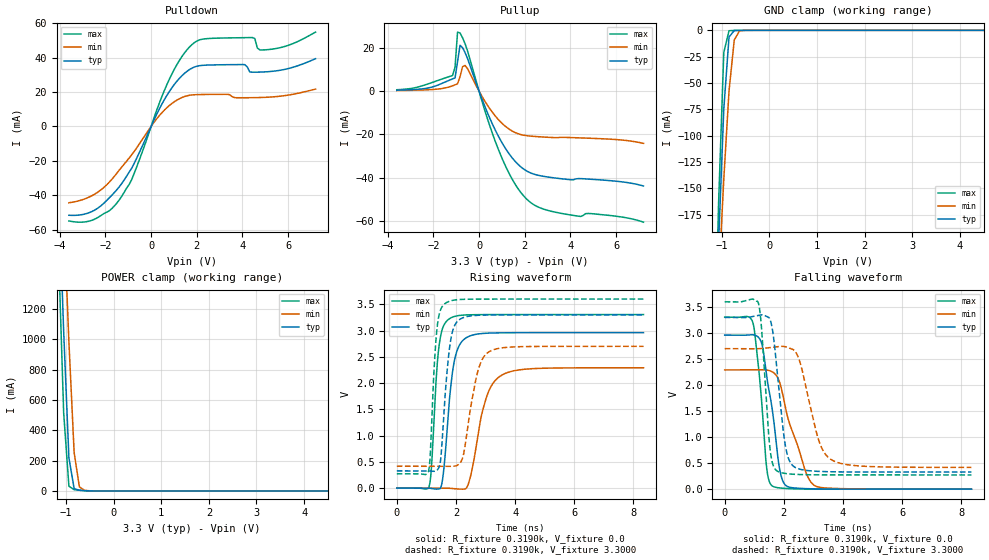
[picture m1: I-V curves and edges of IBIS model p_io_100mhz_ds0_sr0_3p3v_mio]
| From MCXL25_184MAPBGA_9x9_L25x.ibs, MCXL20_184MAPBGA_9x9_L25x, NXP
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[Model] p_io_100mhz_ds0_sr0_3p3v_mio
|   Model p_io_100mhz_ds0_sr0_3p3v_mio
| This model was characterised for following simulation conditions:
| External (pad) voltage:
|   - Typ: 3.3V,   - Min: 2.7V,   - Max: 3.6V
| Library cells for typ/min/max conditions are connected as defined below:
|  pad - External Pad
|  ipp_do_lv - Core Input
|  ipp_obe_lv - Output Buffer Enable
|  IOGC - NC
|  REFH3V3 - REFH3V3
|  REFL3V3 - REFL3V3
|  ZI - NC
|  abut_ncal_vddio[1] - vddio
|  abut_ncal_vddio[2] - vddio
|  abut_ncal_vddio[3] - vssio
|  abut_ncal_vddio[4] - vddio
|  abut_ncal_vddio[5] - vddio
|  abut_ncal_vddio[6] - vssio
|  abut_pcal_vddio[1] - vssio
|  abut_pcal_vddio[2] - vssio
|  abut_pcal_vddio[3] - vddio
|  abut_pcal_vddio[4] - vssio
|  abut_pcal_vddio[5] - vssio
|  abut_pcal_vddio[6] - vddio
|  ipp_do_1p8v - ipp_do_1p8v
|  ipp_dse_lv - 0
|  ipp_eftd_lv - NC
|  ipp_ina_mux_vddio - NC
|  ipp_ina_mux_vddio[0] - NC
|  ipp_ina_mux_vddio[1] - NC
|  ipp_ina_r0_vddio - NC
|  ipp_ina_r0a_vddio - NC
|  ipp_ina_r0b_vddio - NC
|  ipp_ina_r0c_vddio - NC
|  ipp_ina_r0d_vddio - NC
|  ipp_ina_r0e_vddio - NC
|  ipp_ina_r0f_vddio - NC
|  ipp_ina_r300_vddio - NC
|  ipp_ina_r300a_vddio - NC
|  ipp_ina_r300b_vddio - NC
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Model_type I/O
Polarity   Non-Inverting
Enable   Active-High
Vinl =   0.9900V
Vinh =   2.3100V
Vmeas =  1.6500V
Cref =   30.0000pF
Rref =   1.0000M
Vref =   3.3000V
C_comp   1.3235pF   1.2640pF   1.4076pF
|C_comp_pullup   0.6739pF   0.7056pF   0.6519pF
|C_comp_pulldown   0.5816pF   0.6344pF   0.5434pF
[Model Spec]
| variable   typ   min   max
Vinh   2.3100V   1.8900V   2.5200V
Vinl   0.9900V   0.8100V   1.0800V
[Temperature Range]   25.0000   0.1250k   -40.0000
[Voltage Range]   3.3000V   2.7000V   3.6000V
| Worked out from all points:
|   slope of the pulldown table from 0 to 0.495 V, typ, clamps not added: 36.6 ohm
|   slope of the pullup table from 0 to 0.495 V, typ, clamps not added: 37.7 ohm
|   GND clamp passes 1 mA (typ) near -0.75 V on its own axis
|   POWER clamp passes 1 mA (typ) near -0.55 V on its own axis
|   rising waveform, R_fixture 0.3190k, V_fixture 0.0: 20-80 % time 299ps typ, 517ps min, 214ps max; typ from 0 V to 2.96 V
|   rising waveform, R_fixture 0.3190k, V_fixture 3.3000: 20-80 % time 255ps typ, 423ps min, 184ps max; typ from 0.328 V to 3.3 V
|   falling waveform, R_fixture 0.3190k, V_fixture 0.0: 20-80 % time 427ps typ, 707ps min, 290ps max; typ from 2.96 V to 0 V
|   falling waveform, R_fixture 0.3190k, V_fixture 3.3000: 20-80 % time 330ps typ, 583ps min, 237ps max; typ from 3.3 V to 0.329 V
[Pulldown]
|Voltage   I(typ)   I(min)   I(max)
-3.6V     -51.52mA   -44.27mA   -54.81mA
-2.5V     -48.75mA   -39.51mA   -53.96mA
-1.4V     -35.12mA   -25.45mA   -42.73mA
-850mV    -24.27mA   -16.41mA   -30.84mA
800mV     20.29mA    12.16mA    27.43mA
1.35V     29.44mA    16.78mA    40.57mA
1.9V      34.5mA     18.39mA    48.67mA
4.1V      35.87mA    16.66mA    51.51mA
4.43V     31.5mA     16.69mA    51.59mA
4.65V     31.5mA     16.75mA    45.53mA
5.09V     31.75mA    16.96mA    44.55mA
7.2V      39.3mA     21.67mA    54.74mA
[Pullup]
|Voltage   I(typ)   I(min)   I(max)
-3.6V     391.8uA    234.9uA    605.7uA
-1.16V    5.604mA    2.419mA    7.14mA
-1.05V    6.055mA    2.871mA    11mA
-940mV    13.56mA    3.339mA    27.24mA
-830mV    21.15mA    6.685mA    26.82mA
-720mV    20.05mA    11.26mA    24.61mA
-610mV    17.74mA    11.81mA    21.86mA
820mV     -20.29mA   -12.86mA   -26.23mA
1.48V     -31.23mA   -18.63mA   -41.23mA
2.03V     -36.57mA   -20.53mA   -49.31mA
3.46V     -40.33mA   -21.49mA   -56.22mA
7.2V      -43.87mA   -24.17mA   -60.58mA
[GND_clamp]
|Voltage   I(typ)   I(min)   I(max)
-3.6V     -4.134A    -3.035A    -5.609A
-1.18V    -349.4mA   -343.6mA   -365.7mA
-1.07V    -202.9mA   -239.3mA   -165.2mA
-960mV    -74.83mA   -141.5mA   -21.03mA
-850mV    -6.389mA   -57.64mA   -383.3uA
-740mV    -222.1uA   -9.174mA   -124.1uA
-630mV    -55.93uA   -558.9uA   -58.07uA
7.2V      0A         0A         0A
[POWER_clamp]
|Voltage   I(typ)   I(min)   I(max)
-3.6V     24.54A     22.33A     26.93A
-1.16V    2.046A     2.721A     1.599A
-1.05V    1.052A     1.847A     514.4mA
-940mV    218.6mA    981.8mA    31.16mA
-830mV    15.1mA     252.4mA    8.462mA
-720mV    4.281mA    26.81mA    4.453mA
-610mV    1.717mA    3.626mA    1.66mA
7.2V      0A         0A         0A
[Ramp]
| variable   typ   min   max
dV/dt_r  1.7763/0.2988n   1.3750/0.5172n   1.9832/0.2140n
dV/dt_f  1.7829/0.3304n   1.3692/0.5829n   1.9962/0.2366n
R_load = 0.3190k
[Rising Waveform]
R_fixture= 0.3190k
V_fixture= 0.0
V_fixture_min= 0.0
V_fixture_max= 0.0
|time   V(typ)   V(min)   V(max)
0s        2.902nV    250nV      9.459nV
1.086ns   -976.7uV   -29.66uV   18.83mV
1.414ns   -15.5mV    651.1uV    2.638V
1.567ns   247.8mV    1.45mV     3.071V
1.766ns   1.596V     -2.144mV   3.22V
2.173ns   2.772V     -19.8mV    3.292V
2.455ns   2.894V     144.2mV    3.3V
3.05ns    2.95V      1.761V     3.304V
3.542ns   2.957V     2.149V     3.305V
8.34ns    2.961V     2.292V     3.305V
[Rising Waveform]
R_fixture= 0.3190k
V_fixture= 3.3000
V_fixture_min= 2.7000
V_fixture_max= 3.6000
|time   V(typ)   V(min)   V(max)
0s        328.4mV    417.4mV    273mV
1.073ns   327.9mV    417.3mV    324.4mV
1.356ns   339mV      417.7mV    3.019V
1.484ns   549.3mV    418.3mV    3.402V
1.64ns    1.817V     417.6mV    3.518V
1.974ns   3.118V     421.1mV    3.583V
2.25ns    3.247V     626.3mV    3.595V
2.767ns   3.292V     2.277V     3.599V
3.119ns   3.297V     2.597V     3.6V
8.34ns    3.3V       2.7V       3.6V
[Falling Waveform]
R_fixture= 0.3190k
V_fixture= 0.0
V_fixture_min= 0.0
V_fixture_max= 0.0
|time   V(typ)   V(min)   V(max)
0s        2.961V     2.292V     3.305V
954.1ps   2.967V     2.291V     3.197V
1.243ns   2.815V     2.294V     1.731V
1.42ns    2.166V     2.29V      403.1mV
1.604ns   1.548V     2.256V     63.43mV
1.828ns   486.1mV    2.1V       25.24mV
1.982ns   134.6mV    1.766V     16.49mV
2.726ns   10.64mV    351.6mV    2.556mV
3.05ns    5.57mV     66.35mV    1.221mV
8.34ns    83.62uV    191.3uV    53.48uV
[Falling Waveform]
R_fixture= 0.3190k
V_fixture= 3.3000
V_fixture_min= 2.7000
V_fixture_max= 3.6000
|time   V(typ)   V(min)   V(max)
0s        3.3V       2.7V       3.6V
1.141ns   3.342V     2.699V     3.572V
1.245ns   3.351V     2.703V     3.102V
1.533ns   3.259V     2.721V     770.1mV
1.769ns   2.279V     2.737V     349.2mV
2.06ns    805.8mV    2.736V     300.7mV
2.402ns   411.8mV    2.631V     284mV
3.171ns   341.9mV    951.9mV    274.9mV
3.588ns   334.4mV    572.4mV    273.9mV
8.34ns    328.6mV    418.1mV    273.1mV
